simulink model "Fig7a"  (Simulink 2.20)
settings: Solver=ode45  StartTime=0.0  StopTime=1  MaxStep=.001  RelTol=1e-3  AbsTol=1e-6

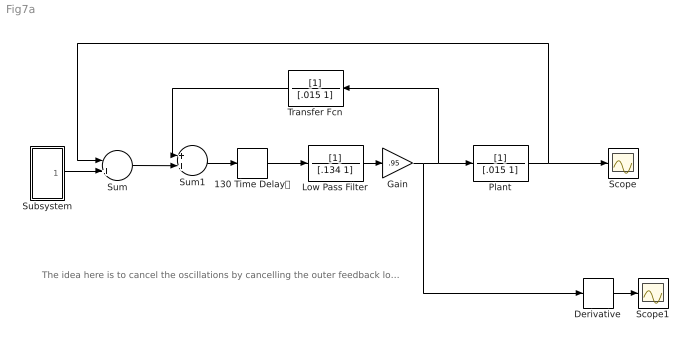
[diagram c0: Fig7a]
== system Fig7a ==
  note: The idea here is to cancel the oscillations by cancelling the outer feedback loop with a matched inner feedback loop Now gain has to be .95 so the only thing that is really a free parameter is the low-pass element in the middle This is the Young anf Yasui basee model presented by robinson in figure 7a, it includes a realistic plant, unlike the original
  130 Time Delay : TransportDelay  DelayTime=.130  InitialInput=0  BufferSize=1024
  Derivative : Derivative
  Gain : Gain  Gain=.95
  Low Pass Filter : TransferFcn  Numerator=[1]  Denominator=[.134 1]
  Plant : TransferFcn  Numerator=[1]  Denominator=[.015 1]
  Scope : Scope
  Scope1 : Scope
  Subsystem : Subsystem
  Sum : Sum  Inputs=-+
  Sum1 : Sum  Inputs=++
  Transfer Fcn : TransferFcn  Orientation=left  Numerator=[1]  Denominator=[.015 1]
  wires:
  Low Pass Filter/1 -> Gain/1
  Plant/1 -> Sum/1, Scope/1
  130 Time Delay/1 -> Low Pass Filter/1
  Sum1/1 -> 130 Time Delay/1
  Transfer Fcn/1 -> Sum1/1
  Sum/1 -> Sum1/2
  Derivative/1 -> Scope1/1
  Gain/1 -> Plant/1, Transfer Fcn/1, Derivative/1
  Subsystem/1(Out1) -> Sum/2

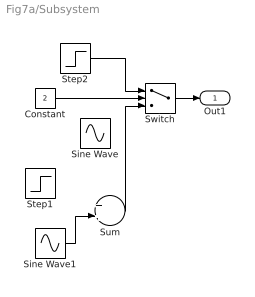
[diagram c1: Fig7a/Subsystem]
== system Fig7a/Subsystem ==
  Constant : Constant  Value=2
  Sine Wave : Sin  Amplitude=10  Frequency=10*pi*2  Phase=0  SampleTime=0
  Sine Wave1 : Sin  Amplitude=8  Frequency=6*pi*2  Phase=0  SampleTime=0
  Step1 : Step  Time=.1  Before=0  After=20
  Step2 : Step  Time=.1  Before=0  After=20
  Sum : Sum  Inputs=++
  Switch : Switch  Threshold=1
  Out1 : Outport  Port=1  InitialOutput=0
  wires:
  Constant/1 -> Switch/2
  Switch/1 -> Out1/1
  Sine Wave1/1 -> Sum/2
  Sum/1 -> Switch/3
  Step2/1 -> Switch/1
